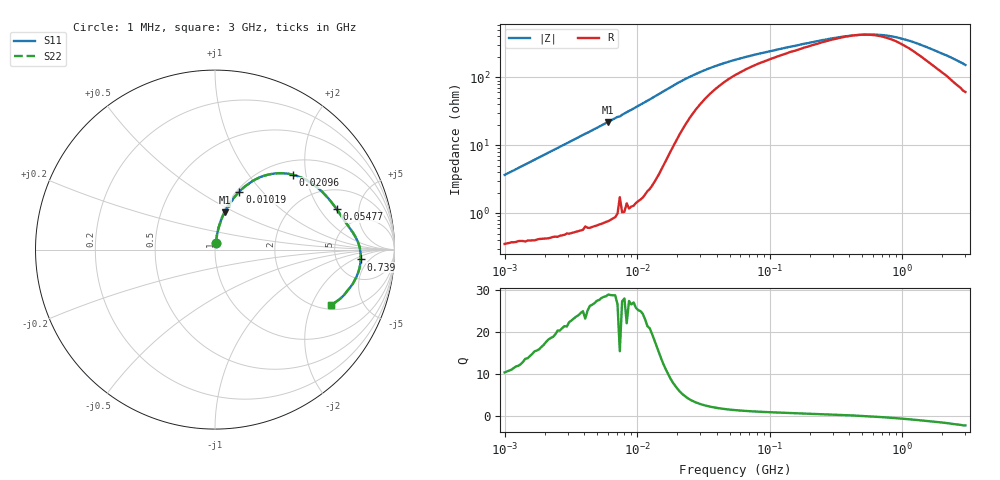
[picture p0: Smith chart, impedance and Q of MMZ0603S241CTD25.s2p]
! S-Parameter Data Generated by TDK Corporation
! Copyright(C) 2025 TDK Corporation.
! All Rights Reserved.
! TDK P/N: MMZ0603S241CTD25 (Chip Bead)
! Property: |Z|=240ohm at 100MHz
! Size(LxWxT): 0.6x0.3x0.3mm
! Model Type: s2p (Touchstone File Format Version 1.0)
! Frequency: DC=Yes Start=1MHz Stop=3000MHz 202points Log-sweep
! Model Generated on Feb. 6, 2025
! Terms and conditions regarding TDK Simulation Models:
! 1)This simulation model is being provided solely for informational
!  purposes. Please refer to the specifications of the products in
!  terms of detailed characteristics of such products.
! 2)In no event shall TDK Corporation of any of its subsidiaries be
!  liable for any loss or damage arising, directly or indirectly,
!  from any information contained in this simulation model, including,
!  but not limited to loss or damages arising from any inaccuracies,
!  omissions or errors in connection with such information.
! 3)Any and all copyrights on this simulation model are owned by
!  TDK Corporation.  Duplication or redistribution of this simulation
!  model without prior written permission from TDK Corporation
!  is prohibited.
! 4)This simulation model is subject to any modification or change
!  without any prior notice.
! 5)Neither TDK Corporation nor any of its subsidiaries shall make any
!  warranty, express or implied, including but not limited to the
!  correctness, implied warranties of merchantability and fitness for
!  a particular purpose with respect to this simulation models.
! 6)The use of this simulation model shall be deemed to have consented
!  to the terms and conditions hereof.
! Port Assignments:
!  1 ---@@@--- 2
! Applicable Conditions:
!  Temperature = 25 degC
!  DC Bias Current = 0 A
!  Small Signal Operation
# Hz S MA R 50
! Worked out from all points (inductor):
!   201 points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, 1 MHz to 3 GHz, reference 50 ohm
!   read as one part in series: L = 580 nH near 1.041 MHz
!   highest Q = 28.7 at 6.058 MHz (marker M1), where L = 582 nH
!   self-resonance near 473.3 MHz
!   S11 on the Smith chart (normalised r, x): 1 MHz: 1.01, +0.07; 10.19 MHz: 1.03, +0.76; 20.96 MHz: 1.29, +1.69; 54.77 MHz: 3.16, +2.91; 739 MHz: 8.80, -2.87; 3 GHz: 2.22, -2.79
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1000000  0.03658 82.4  0.9958 -2.1  0.9958 -2.1  0.03658 82.4
2139570  0.07739 82.4  0.9928 -4.4  0.9928 -4.4  0.07739 82.4
3900413  0.14 79.7  0.9846 -8.0  0.9846 -8.0  0.14 79.7
6058321  0.2147 75.6  0.9693 -12.4  0.9693 -12.4  0.2147 75.6
7400828  0.2527 71.7  0.9513 -14.6  0.9513 -14.6  0.2527 71.7
1.019448e7  0.3506 67.2  0.9227 -20.5  0.9227 -20.5  0.3506 67.2
1.461624e7  0.4822 57.5  0.8448 -28.8  0.8448 -28.8  0.4822 57.5
1.785516e7  0.5551 50.1  0.7717 -33.5  0.7717 -33.5  0.5551 50.1
2.095589e7  0.6019 43.8  0.7026 -36.4  0.7026 -36.4  0.6019 43.8
2.559965e7  0.6436 36.5  0.6156 -38.4  0.6156 -38.4  0.6436 36.5
3.254976e7  0.6753 29.1  0.5257 -38.7  0.5257 -38.7  0.6753 29.1
5.477226e7  0.7139 18.4  0.3939 -35.0  0.3939 -35.0  0.7139 18.4
9.593103e7  0.7431 11.9  0.3126 -29.2  0.3126 -29.2  0.7431 11.9
2.136344e8  0.7814 5.7  0.2358 -19.4  0.2358 -19.4  0.7814 5.7
4.219165e8  0.8062 0.9  0.1943 -3.7  0.1943 -3.7  0.8062 0.9
5.81181e8  0.8122 -1.7  0.1896 7.2  0.1896 7.2  0.8122 -1.7
7.38967e8  0.814 -3.9  0.1958 16.3  0.1958 16.3  0.814 -3.9
8.005644e8  0.8141 -4.7  0.1999 19.4  0.1999 19.4  0.8141 -4.7
1.147801e9  0.8088 -8.7  0.2353 31.5  0.2353 31.5  0.8088 -8.7
1.645649e9  0.7913 -13.9  0.2998 39.3  0.2998 39.3  0.7913 -13.9
2.359433e9  0.7576 -20.2  0.3893 42.1  0.3893 42.1  0.7576 -20.2
3e9  0.7146 -25.5  0.4692 40.9  0.4692 40.9  0.7146 -25.5
